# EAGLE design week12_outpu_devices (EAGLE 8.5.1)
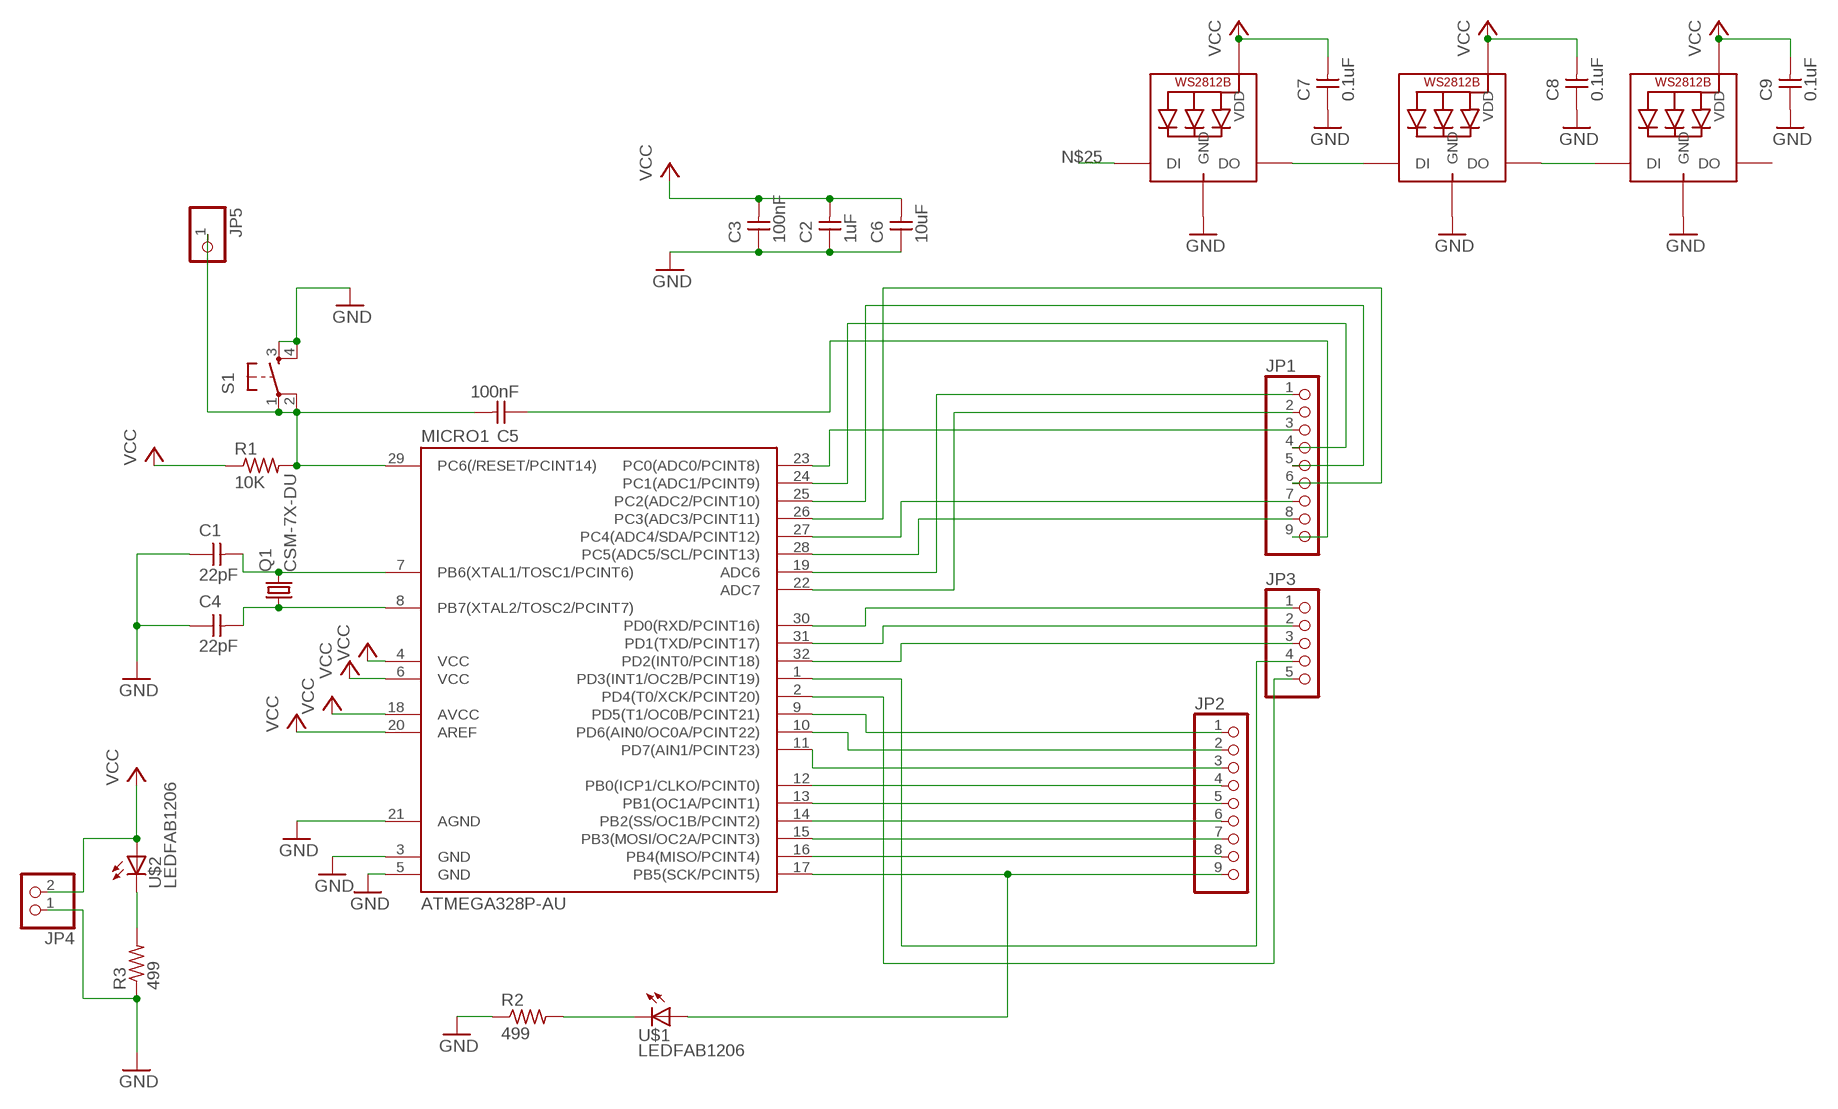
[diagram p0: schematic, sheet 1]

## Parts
C1  22pF  CAP-UNPOLARIZEDFAB  [C1206FAB]
C2  1uF  CAP-UNPOLARIZEDFAB  [C1206FAB]
C3  100nF  CAP-UNPOLARIZEDFAB  [C1206FAB]
C4  22pF  CAP-UNPOLARIZEDFAB  [C1206FAB]
C5  100nF  CAP-UNPOLARIZEDFAB  [C1206FAB]
C6  10uF  CAP-UNPOLARIZEDFAB  [C1206FAB]
C7  0.1uF  CAP-UNPOLARIZEDFAB  [C1206FAB]
C8  0.1uF  CAP-UNPOLARIZEDFAB  [C1206FAB]
C9  0.1uF  CAP-UNPOLARIZEDFAB  [C1206FAB]
JP1  PINHD-1X9  [1X09]
JP2  PINHD-1X9  [1X09]
JP3  PINHD-1X5  [1X05]
JP4  PINHD-1X2  [1X02]
JP5  PINHD-1X1  [1X01]
LED1  WS2812B_5050N  [WS2812B-NARROW]
LED2  WS2812B_5050N  [WS2812B-NARROW]
LED3  WS2812B_5050N  [WS2812B-NARROW]
MICRO1  ATMEGA328P-AU  ATMEGA48/88/168-AU  [TQFP32-08]
Q1  CSM-7X-DU  [CSM-7X-DU]
R1  10K  RES-US1206FAB  [R1206FAB]
R2  499  RES-US1206FAB  [R1206FAB]
R3  499  RES-US1206FAB  [R1206FAB]
S1  6MM_SWITCH6MM_SWITCH  [6MM_SWITCH]
U$1  LEDFAB1206  [LED1206FAB]
U$2  LEDFAB1206  [LED1206FAB]

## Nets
GND: C1.1 C2.1 C3.1 C4.1 C6.1 C7.1 C8.1 C9.1 JP4.1 LED1.3-GND(GND) LED2.3-GND(GND) LED3.3-GND(GND) MICRO1.3(GND) MICRO1.5(GND) MICRO1.21(AGND) R2.1 R3.1 S1.3(S) S1.4(S1)
N$1: C1.2 MICRO1.7(PB6(XTAL1/TOSC1/PCINT6)) Q1.2
N$2: C4.2 MICRO1.8(PB7(XTAL2/TOSC2/PCINT7)) Q1.1
N$3: JP2.9 MICRO1.17(PB5(SCK/PCINT5)) U$1.1(A)
N$4: JP2.8 MICRO1.16(PB4(MISO/PCINT4))
N$5: JP2.7 MICRO1.15(PB3(MOSI/OC2A/PCINT3))
N$6: JP2.6 MICRO1.14(PB2(SS/OC1B/PCINT2))
N$7: JP2.5 MICRO1.13(PB1(OC1A/PCINT1))
N$8: JP2.4 MICRO1.12(PB0(ICP1/CLKO/PCINT0))
N$9: JP2.3 MICRO1.11(PD7(AIN1/PCINT23))
N$10: JP2.2 MICRO1.10(PD6(AIN0/OC0A/PCINT22))
N$11: JP2.1 MICRO1.9(PD5(T1/OC0B/PCINT21))
N$12: JP3.5 MICRO1.2(PD4(T0/XCK/PCINT20))
N$13: JP3.4 MICRO1.1(PD3(INT1/OC2B/PCINT19))
N$14: JP3.1 MICRO1.30(PD0(RXD/PCINT16))
N$15: JP3.2 MICRO1.31(PD1(TXD/PCINT17))
N$16: JP3.3 MICRO1.32(PD2(INT0/PCINT18))
N$17: R2.2 U$1.2(C)
N$18: R3.2 U$2.2(C)
N$19: C5.1 JP1.9
N$20: JP1.3 MICRO1.23(PC0(ADC0/PCINT8))
N$21: JP1.4 MICRO1.24(PC1(ADC1/PCINT9))
N$22: JP1.5 MICRO1.25(PC2(ADC2/PCINT10))
N$23: JP1.6 MICRO1.26(PC3(ADC3/PCINT11))
N$24: JP1.7 MICRO1.27(PC4(ADC4/SDA/PCINT12))
N$25: JP1.8 LED1.4-DIN(DI) MICRO1.28(PC5(ADC5/SCL/PCINT13))
N$26: JP1.1 MICRO1.19(ADC6)
N$27: JP1.2 MICRO1.22(ADC7)
N$28: LED1.2-DOUT(DO) LED2.4-DIN(DI)
N$29: C5.2 JP5.1 MICRO1.29(PC6(/RESET/PCINT14)) R1.2 S1.1(P) S1.2(P1)
N$30: LED2.2-DOUT(DO) LED3.4-DIN(DI)
VCC: C2.2 C3.2 C6.2 C7.2 C8.2 C9.2 JP4.2 LED1.1-VDD(VDD) LED2.1-VDD(VDD) LED3.1-VDD(VDD) MICRO1.4(VCC) MICRO1.6(VCC) MICRO1.18(AVCC) MICRO1.20(AREF) R1.1 U$2.1(A)
Unconnected: LED3.2-DOUT(DO)

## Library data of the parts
C1-C9 = fab:CAP-UNPOLARIZED
JP1 JP2 = pinhead:PINHD-1X9: PIN HEADER
JP3 = pinhead:PINHD-1X5: PIN HEADER
JP4 = pinhead:PINHD-1X2: PIN HEADER
JP5 = pinhead:PINHD-1X1: PIN HEADER
LED1-LED3 = adafruit:WS2812B
MICRO1 = atmega8:ATMEGA48/88/168
Q1 = crystal-2:CSM-7X-DU: SMD CRYSTAL; OC_FARNELL: unknown; OC_NEWARK: unknown
R1-R3 = fab:RES-US: Resistor (US Symbol)
S1 = fab:6MM_SWITCH: OMRON SWITCH
U$1 U$2 = fab:LED: LED

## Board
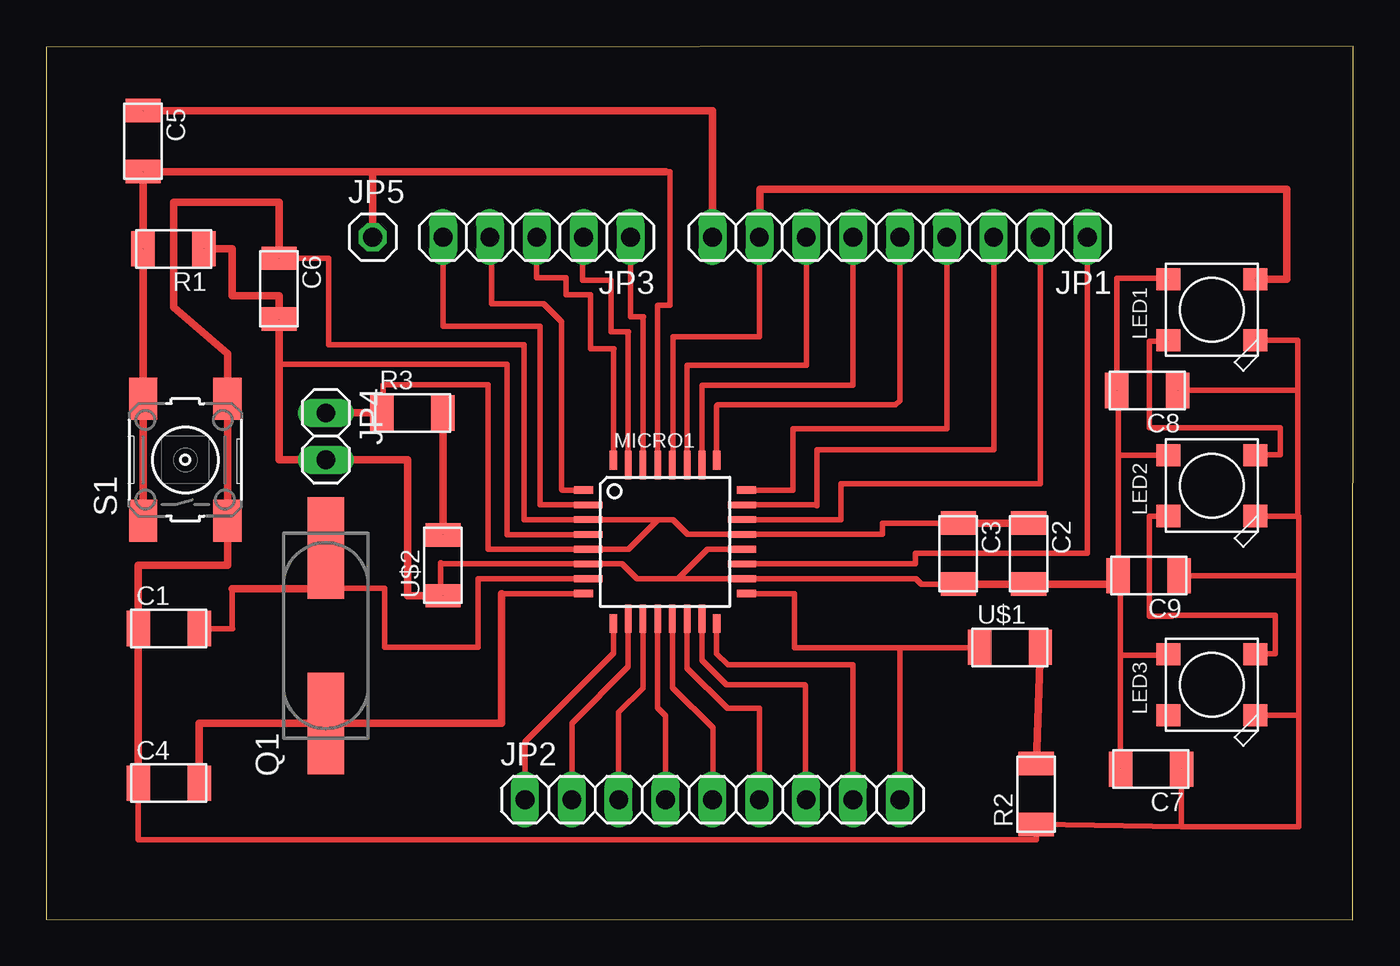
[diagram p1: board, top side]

Size 70.87 x 47.34 mm. Coordinates in mm from the lower left corner, seen from the top.
Outline: 0,0.03 70.84,0 70.87,47.34 0,47.28 0,0.03
Copper layers (1*16): Top 0.035mm / dielectric 1.5mm / Bottom 0.035mm
Design rules "default *": minimum track width 6mil, minimum drill 0.35mm, track to track 0.4mm, track to pad 0.4mm, pad to pad 0.4mm, via to via 0.4mm, smd to smd 0.4mm, copper to edge 40mil, drill to drill 6mil, minimum pad ring 10mil, minimum via ring 8mil, stop-mask expansion 4mil, vias tented up to drill 0mil, thermal gap 10mil

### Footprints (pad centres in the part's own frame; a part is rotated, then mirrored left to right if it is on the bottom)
C1206FAB = smd 1.27 x 1.905: 1 -1.651,0; 2 1.651,0
1X09 = drill 1.016 long: 1 -10.16,0; 2 -7.62,0; 3 -5.08,0; 4 -2.54,0; 5 0,0; 6 2.54,0; 7 5.08,0; 8 7.62,0; 9 10.16,0
1X05 = drill 1.016 long: 1 -5.08,0; 2 -2.54,0; 3 0,0; 4 2.54,0; 5 5.08,0
1X02 = drill 1.016 long: 1 -1.27,0; 2 1.27,0
1X01 = drill 1.016 octagon: 1 0,0
WS2812B-NARROW = smd 1.3 x 1.2: 1-VDD 2.35,-1.65; 2-DOUT 2.35,1.65; 3-GND -2.35,1.65; 4-DIN -2.35,-1.65
TQFP32-08 = smd 1.016 x 0.406: 1 -4.42,2.8; 8 -4.42,-2.8; 17 4.42,-2.8; 24 4.42,2.8 | smd 1.524 x 0.356: 2 -4.166,2; 3 -4.166,1.2; 4 -4.166,0.4; 5 -4.166,-0.4; 6 -4.166,-1.2; 7 -4.166,-2; 18 4.166,-2; 19 4.166,-1.2; 20 4.166,-0.4; 21 4.166,0.4; 22 4.166,1.2; 23 4.166,2 | smd 0.406 x 1.016: 9 -2.8,-4.42; 16 2.8,-4.42; 25 2.8,4.42; 32 -2.8,4.42 | smd 0.356 x 1.524: 10 -2,-4.166; 11 -1.2,-4.166; 12 -0.4,-4.166; 13 0.4,-4.166; 14 1.2,-4.166; 15 2,-4.166; 26 2,4.166; 27 1.2,4.166; 28 0.4,4.166; 29 -0.4,4.166; 30 -1.2,4.166; 31 -2,4.166
CSM-7X-DU = smd 5.5 x 2: 1 -4.75,0; 2 4.75,0
R1206FAB = smd 1.27 x 1.905: 1 -1.651,0; 2 1.651,0
6MM_SWITCH = smd 2.286 x 1.524: 1 -3.302,2.286; 2 3.302,2.286; 3 -3.302,-2.286; 4 3.302,-2.286
LED1206FAB = smd 1.27 x 1.905: 1 -1.651,0; 2 1.651,0

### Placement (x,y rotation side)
C1  6.65,15.77 0 top
C2  53.26,19.84 270 top
C3  49.45,19.84 270 top
C4  6.65,7.39 0 top
C5  5.26,42.19 270 top
C6  12.62,34.19 270 top
C7  59.89,8.15 180 top
C8  59.69,28.68 180 top
C9  59.77,18.64 180 top
JP1  46.28,36.98 180 top
JP2  36.12,6.5 0 top
JP3  26.59,36.98 180 top
JP4  15.16,26.19 270 top
JP5  17.7,36.98 0 top
LED1  63.2,33.05 180 top
LED2  63.2,23.52 180 top
LED3  63.2,12.73 180 top
MICRO1  33.55,20.47 0 top
Q1  15.16,15.39 90 top
R1  6.91,36.35 180 top
R2  53.67,6.81 90 top
R3  19.86,27.46 0 top
S1  7.54,24.92 90 top
U$1  52.25,14.76 0 top
U$2  21.51,19.2 90 top

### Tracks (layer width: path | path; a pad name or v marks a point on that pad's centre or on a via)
GND  (4 unrouted)
  Top 0.305: C4.1 5,4.32 53.67,4.32 R2.1 61.54,5.03 | 61.54,5.03 C7.1 | 61.54,5.03 67.89,5.03 67.89,11.08 | 67.89,21.79 67.89,21.87 LED2.3-GND | 67.89,21.79 67.89,18.64 | 67.89,18.64 67.89,11.08 | LED3.3-GND 67.89,11.08 | C9.1 67.89,18.64 | LED1.3-GND 67.84,31.4 67.84,28.68 | C8.1 67.84,28.68 | 67.89,21.79 67.84,21.79 67.84,28.68 | C3.1 45.34,21.49 45.34,20.87 MICRO1.21 34.78,20.87 33.98,21.67 33.15,21.67 | C6.1 15.32,35.84 15.32,31.17 25.91,31.17 25.91,21.67 MICRO1.3 33.15,21.67 | R3.1 18.26,27.46 18.26,28.98 23.95,28.98 23.95,20.07 MICRO1.5 31.58,20.07 33.15,21.64 33.15,21.67
  Top 0.406: JP4.1 R3.1 | C4.1 C1.1 5,19.2 9.83,19.2 S1.3 S1.4 9.86,30.66 6.91,33.17 6.91,38.89 12.62,38.89 C6.1 | C3.1 C2.1
N$1
  Top 0.305: 15.16,17.93 15.16,17.96 18.34,17.96 18.34,14.76 23.42,14.76 23.42,18.47 MICRO1.7 | 10.08,17.93 10.08,15.77 | 10.08,15.77 10.11,15.77 | 10.08,15.77 C1.2
  Top 0.406: 10.08,17.93 15.16,17.93 Q1.2
N$2
  Top 0.305: MICRO1.8 24.69,17.67
  Top 0.406: 24.69,17.67 24.69,10.64 Q1.1 8.31,10.64 C4.2
N$3
  Top 0.305: U$1.1 50.6,14.73 46.28,14.73 | 46.28,14.73 40.56,14.73 40.56,17.67 MICRO1.17 | JP2.9 46.28,14.73
N$4
  Top 0.305: MICRO1.16 36.35,14.42 36.96,13.82 43.74,13.82 JP2.8
N$5
  Top 0.305: MICRO1.15 35.55,14.05 36.88,12.73 41.12,12.73 41.17,12.67 41.17,6.53 JP2.7
N$6
  Top 0.305: MICRO1.14 34.75,13.63 36.93,11.46 38.66,11.46 JP2.6
N$7
  Top 0.305: MICRO1.13 33.95,12.58 36.14,10.39 36.14,6.53 JP2.5
N$8
  Top 0.305: MICRO1.12 33.15,11.47 33.58,11.05 JP2.4
N$9
  Top 0.305: MICRO1.11 32.35,12.54 31.04,11.23 JP2.3
N$10
  Top 0.305: MICRO1.10 31.55,13.7 28.5,10.64 JP2.2
N$11
  Top 0.305: MICRO1.9 30.75,14.45 25.96,9.65 JP2.1
N$12
  Top 0.305: JP3.5 21.51,32.16 26.77,32.16 26.77,22.47 MICRO1.2
N$13
  Top 0.305: JP3.4 24.16,36.88 24.16,33.38 26.98,33.38 27.94,32.41 27.94,23.32 27.99,23.27 28,23.27 MICRO1.1
N$14
  Top 0.305: JP3.1 31.67,32.66 32.38,32.66 32.35,32.64 MICRO1.30
N$15
  Top 0.305: JP3.2 29.08,36.98 29.08,34.65 30.63,34.65 30.63,31.85 31.58,31.85 31.55,31.83 MICRO1.31
N$16
  Top 0.305: JP3.3 26.59,34.77 28.19,34.77 28.19,33.86 29.52,33.86 29.52,30.94 30.78,30.94 30.75,30.91 MICRO1.32
N$17
  Top 0.406: U$1.2 R2.2
N$18  (1 unrouted)
  Top 0.406: R3.2 | R3.2 U$2.2
N$19  (1 unrouted)
  Top 0.406: JP1.9 36.12,43.84 C5.1
N$20
  Top 0.305: JP1.3 51.38,36.98 51.38,25.48 41.78,25.48 41.78,22.43 41.74,22.47 MICRO1.23
N$21
  Top 0.305: JP1.4 48.82,26.59 40.49,26.59 40.49,23.27 MICRO1.24
N$22
  Top 0.305: MICRO1.25 36.35,27.82 36.42,27.89 46.05,27.89 46.28,28.12 JP1.5
N$23
  Top 0.305: JP1.6 43.74,28.96 35.58,28.96 35.55,28.93 MICRO1.26
N$24
  Top 0.305: JP1.7 41.22,36.98 41.22,30.05 34.78,30.05 34.75,30.02 MICRO1.27
N$25  (1 unrouted)
  Top 0.152: 38.85,36.54 38.66,36.35
  Top 0.305: 38.66,36.65 38.66,31.6 33.98,31.6 33.98,24.66 MICRO1.28
  Top 0.406: 38.66,36.35 38.66,36.65 JP1.8 38.71,36.98 38.71,39.57 67.26,39.57 67.26,34.7 LED1.4-DIN
N$26
  Top 0.305: 47.12,19.27 47.12,19.35 | 47.12,19.35 47.12,19.86 56.44,19.86 JP1.1 | MICRO1.19 47.03,19.27 47.12,19.35
N$27
  Top 0.305: JP1.2 53.9,23.62 43.08,23.62 43.08,21.67 43.03,21.67 MICRO1.22
N$28  (1 unrouted)
  Top 0.305: LED1.2-DOUT 60.84,31.34 59.79,31.34 59.79,26.64 66.9,26.64 66.9,25.2 65.55,25.2 LED2.4-DIN
N$29  (2 unrouted)
  Top 0.305: 33.58,40.54 33.83,40.54 33.83,33.3 33.18,33.3 33.15,33.27 MICRO1.29
  Top 0.406: S1.1 S1.2 R1.2 | 17.7,40.54 JP5.1 | 33.33,40.54 33.58,40.54 | 33.33,40.54 | 33.33,40.54 17.7,40.54 | R1.2 C5.2 17.7,40.54 | R1.2
N$30
  Top 0.305: LED3.4-DIN 65.55,14.4 66.62,14.4 66.62,16.48 61.06,16.48 | 60.84,16.48 61.06,16.48 | LED2.2-DOUT 59.79,21.87 59.79,16.43 61.06,16.43 61.06,16.48
VCC  (6 unrouted)
  Top 0.305: 49.45,18.47 C3.2 | 12.62,30.1 24.99,30.1 24.99,20.85 29.37,20.85 MICRO1.4 | 34.27,18.47 32.02,18.47 31.22,19.27 MICRO1.6 21.44,19.27 21.39,19.33 21.39,17.68 U$2.1 | 34.27,18.47 MICRO1.18 47.16,18.47 47.45,18.19 49.63,18.19 | MICRO1.20 35.87,20.07 34.27,18.47 | 58.04,18.64 C9.2 | C7.2 58.24,14.33 | 58.24,14.33 58.24,18.64 C9.2 | LED3.1-VDD 60.84,14.33 58.24,14.33 | LED1.1-VDD 60.84,34.75 58.04,34.75 C8.2 58.12,28.68 58.12,25.17 | C9.2 58.12,25.17 | 58.12,25.17 LED2.1-VDD
  Top 0.406: C3.2 49.63,18.19 C2.2 57.66,18.19 C9.2 | C6.2 12.62,30.1 12.62,24.92 JP4.2 19.61,24.92 19.61,17.55 U$2.1 | C6.2 12.62,33.81 10.08,33.81 10.08,36.35 R1.1 | C6.2 | C6.2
